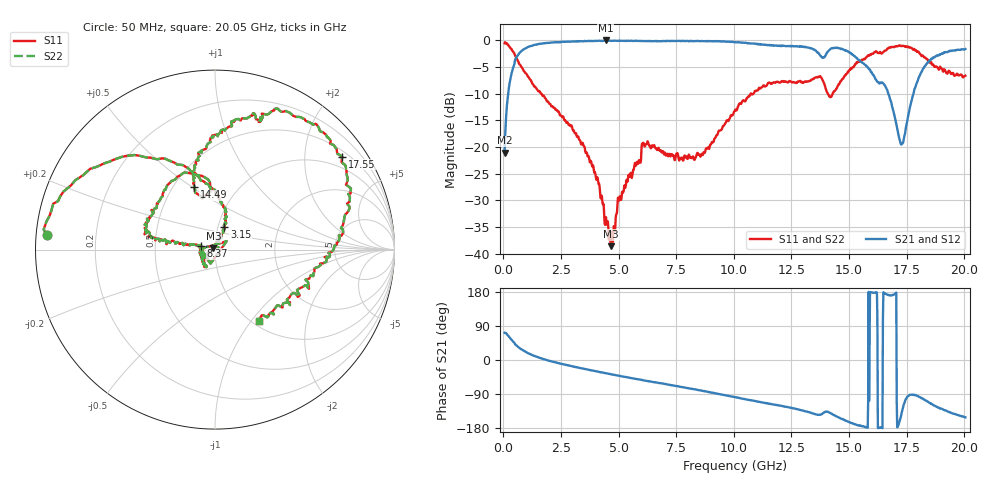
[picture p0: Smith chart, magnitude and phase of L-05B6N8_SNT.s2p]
! P/N: L-05C6N8_SHUNT
! Measured by Marlon
! Sep. 23, 2003
! Measure with a Shunt-through-fixture
#	mhz	s	ma	r	50
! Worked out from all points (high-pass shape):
!   1001 points, 50 MHz to 20.05 GHz, reference 50 ohm
!   highest |S21| = -0.02 dB at 4.43 GHz (marker M1); lowest = -21.0 dB at 50 MHz (marker M2)
!   |S21| within 3 dB of the highest: 584.8 MHz to 13.79 GHz (13.2 GHz wide, 184 % of centre); 18.75 GHz to end of sweep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
!   lowest |S11| = -38.6 dB at 4.67 GHz (marker M3), VSWR 1.02, Z = 49.1 + j0.722 ohm
!   |S11| at or under -10 dB: 1.649 GHz to 10.73 GHz (9.079 GHz wide, 147 % of centre); 10.76 GHz to 10.85 GHz (94.86 MHz wide, 0.878 % of centre); 14.08 GHz to 14.28 GHz (203.1 MHz wide, 1.43 % of centre)
!   |S22| runs from -38.6 to -0.3 dB; largest |S21 - S12| = 0
!   S11 on the Smith chart (normalised r, x): 50 MHz: 0.03, +0.04; 3.15 GHz: 1.07, +0.27; 8.37 GHz: 0.85, +0.04; 14.49 GHz: 0.63, +0.51; 17.55 GHz: 0.65, +2.94; 20.05 GHz: 1.08, -1.09
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50  0.9387 175.0  0.08882 71.8  0.08882 71.8  0.9387 175.0
290  0.8549 152.0  0.4215 57.5  0.4215 57.5  0.8549 152.0
650  0.6275 125.2  0.7396 34.0  0.7396 34.0  0.6275 125.2
1510  0.3346 91.7  0.925 6.9  0.925 6.9  0.3346 91.7
3150  0.1348 67.3  0.9784 -18.8  0.9784 -18.8  0.1348 67.3
3390  0.1057 65.7  0.9832 -21.8  0.9832 -21.8  0.1057 65.7
4430  0.02082 83.3  0.9979 -34.8  0.9979 -34.8  0.02082 83.3
4670  0.01179 141.4  0.989 -37.6  0.989 -37.6  0.01179 141.4
6090  0.1078 -117.6  0.9851 -53.8  0.9851 -53.8  0.1078 -117.6
6730  0.09844 -136.1  0.9791 -60.5  0.9791 -60.5  0.09844 -136.1
8370  0.08246 165.3  0.9849 -78.0  0.9849 -78.0  0.08246 165.3
10050  0.2183 170.7  0.9592 -97.8  0.9592 -97.8  0.2183 170.7
11570  0.3996 167.1  0.9017 -116.0  0.9017 -116.0  0.3996 167.1
13390  0.4294 132.0  0.8376 -140.1  0.8376 -140.1  0.4294 132.0
13970  0.3635 94.2  0.7156 -136.4  0.7156 -136.4  0.3635 94.2
14490  0.3668 108.4  0.8527 -149.9  0.8527 -149.9  0.3668 108.4
15990  0.748 78.2  0.4969 178.0  0.4969 178.0  0.748 78.2
16730  0.8519 67.0  0.3075 171.5  0.3075 171.5  0.8519 67.0
17250  0.8846 48.8  0.1062 -149.6  0.1062 -149.6  0.8846 48.8
17550  0.8777 36.1  0.1905 -95.6  0.1905 -95.6  0.8777 36.1
18570  0.6236 -6.3  0.6733 -115.9  0.6733 -115.9  0.6236 -6.3
20050  0.4664 -57.9  0.8292 -151.3  0.8292 -151.3  0.4664 -57.9
